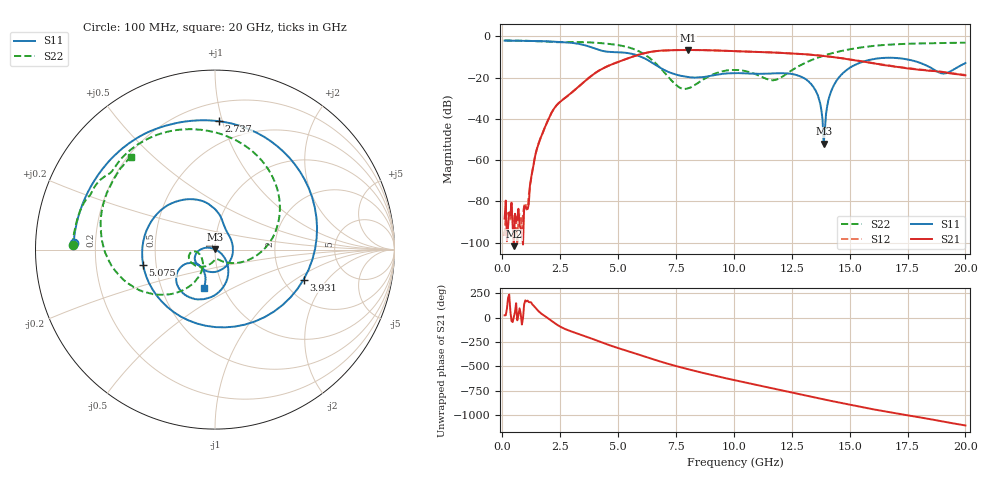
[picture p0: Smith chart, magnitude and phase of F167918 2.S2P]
!  2-Port S-parameters saved by WinCal
! VAR MeasName=S-Parameters (CALIBRATED_DATA) read from VNA (N5242A)
! VAR MeasDate=2016-11-22 10:24:57
! VAR NAME=F167918 2
! VAR FILENAME=F167918 2.S2P
! VAR DATE=2016-11-22 10:24:57
! VAR PHYS_PORTS=1,2
# Hz S DB R 50
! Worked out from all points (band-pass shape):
!   401 points, 100 MHz to 20 GHz, reference 50 ohm
!   highest |S21| = -6.64 dB at 8.01 GHz (marker M1); lowest = -101.8 dB at 498 MHz (marker M2)
!   |S21| within 3 dB of the highest: 5.689 GHz to 13.95 GHz (8.261 GHz wide, 84.1 % of centre)
!   lowest |S11| = -52.1 dB at 13.88 GHz (marker M3), VSWR 1.00, Z = 49.9 + j0.222 ohm
!   |S11| at or under -10 dB: 6.007 GHz to end of sweep
!   |S22| runs from -25.5 to -2.0 dB; largest |S21 - S12| = 0.0051
!   S11 on the Smith chart (normalised r, x): 100 MHz: 0.12, +0.02; 2.737 GHz: 0.33, +0.98; 3.931 GHz: 2.56, -1.18; 5.075 GHz: 0.42, -0.08; 20 GHz: 0.81, -0.37
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1e8  -2.07 177.3  -88.44 22.3  -96.84 28.0  -2.00 178.3
4.98e8  -2.12 166.7  -101.78 7.1  -96.27 19.5  -2.05 171.8
1.04525e9  -2.21 151.8  -83.46 166.3  -83.99 154.0  -2.16 162.8
1.64225e9  -2.33 133.7  -49.70 48.3  -49.64 48.4  -2.41 153.6
2.73675e9  -2.91 88.2  -29.64 -120.3  -29.65 -120.7  -2.78 137.2
3.43325e9  -3.96 37.9  -23.04 -179.8  -23.07 -179.9  -2.81 122.9
3.93075e9  -5.66 -18.7  -18.47 137.3  -18.46 137.4  -3.03 110.6
4.42825e9  -7.29 -89.8  -15.11 93.0  -15.07 92.8  -3.46 96.4
5.075e9  -7.76 -168.3  -12.11 41.0  -12.07 40.5  -4.41 73.7
5.82125e9  -9.22 129.7  -9.15 -15.3  -9.17 -15.8  -6.84 38.0
6.7665e9  -14.85 79.2  -7.01 -87.4  -7.05 -87.6  -14.67 -19.9
8.01025e9  -19.72 26.4  -6.64 -169.7  -6.65 -169.7  -25.26 -86.3
1.005e10  -17.83 -110.0  -7.18 75.7  -7.17 75.8  -16.31 -159.5
1.169175e10  -18.01 -139.4  -7.84 -8.0  -7.82 -8.1  -21.36 -152.1
1.338325e10  -23.84 173.2  -8.97 -94.6  -8.98 -94.4  -11.38 -126.6
1.3632e10  -28.75 164.0  -9.25 -107.2  -9.27 -107.0  -10.32 -130.0
1.388075e10  -52.12 116.0  -9.54 -119.9  -9.54 -119.5  -9.37 -133.7
1.417925e10  -27.39 -32.5  -9.89 -134.9  -9.92 -134.6  -8.38 -138.8
1.4627e10  -18.78 -51.6  -10.60 -157.0  -10.56 -156.7  -7.14 -146.4
1.67165e10  -10.41 -122.4  -14.28 108.7  -14.22 108.9  -4.05 176.7
1.905475e10  -18.10 -132.0  -17.39 11.6  -17.31 11.3  -3.25 143.7
2e10  -12.95 -106.5  -18.91 -27.8  -18.74 -27.9  -3.12 132.0
